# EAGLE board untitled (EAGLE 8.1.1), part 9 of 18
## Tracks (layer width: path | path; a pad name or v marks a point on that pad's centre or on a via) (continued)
S$8777 (continued)
  Bottom 0: 278.09,159.43 277.79,159.54
S$8778
  Bottom 0: 277.79,159.54 277.46,159.56
S$8779
  Bottom 0: 277.46,159.56 277.14,159.49
S$8780
  Bottom 0: 277.14,159.49 276.85,159.34
S$8781
  Bottom 0: 276.85,159.34 276.62,159.12
S$8782
  Bottom 0: 276.62,159.12 276.44,158.85
S$8783
  Bottom 0: 276.44,158.85 276.43,158.81
S$8784
  Bottom 0: 276.43,158.81 271.22,158.81
S$8785
  Bottom 0: 271.22,158.81 271.4,159.02
S$8786
  Bottom 0: 271.4,159.02 271.54,159.32
S$8787
  Bottom 0: 271.54,159.32 271.59,159.64
S$8788
  Bottom 0: 271.59,159.64 271.55,159.94
S$8789
  Bottom 0: 271.55,159.94 276.28,164.67
S$8790
  Bottom 0: 276.28,164.67 276.34,164.73
S$8791
  Bottom 0: 276.34,164.73 276.38,164.81
S$8792
  Bottom 0: 276.38,164.81 276.42,164.89
S$8793
  Bottom 0: 276.42,164.89 276.44,164.98
S$8794
  Bottom 0: 276.44,164.98 276.44,165.07
S$8795
  Bottom 0: 276.44,165.07 276.44,166.09
S$8796
  Bottom 0: 276.44,166.09 282.13,166.09
S$8797
  Bottom 0: 282.13,166.09 282.13,166.06
S$8798
  Bottom 0: 282.13,166.06 282.14,165.99
S$8799
  Bottom 0: 282.14,165.99 282.18,165.92
S$8800
  Bottom 0: 282.18,165.92 282.24,165.86
S$8801
  Bottom 0: 282.24,165.86 282.31,165.82
S$8802
  Bottom 0: 282.31,165.82 282.38,165.81
S$8803
  Bottom 0: 282.38,165.81 284.54,165.81
S$8804
  Bottom 0: 284.54,165.81 284.62,165.82
S$8805
  Bottom 0: 284.62,165.82 284.69,165.86
S$8806
  Bottom 0: 284.69,165.86 284.74,165.92
S$8807
  Bottom 0: 284.74,165.92 284.79,165.99
S$8808
  Bottom 0: 284.79,165.99 284.8,166.06
S$8809
  Bottom 0: 284.8,166.06 284.8,167.26
S$8810
  Bottom 0: 284.8,167.26 284.79,167.34
S$8811
  Bottom 0: 284.79,167.34 284.74,167.41
S$8812
  Bottom 0: 284.74,167.41 284.69,167.47
S$8813
  Bottom 0: 284.69,167.47 284.62,167.51
S$8814
  Bottom 0: 284.62,167.51 284.54,167.52
S$8815
  Bottom 0: 284.54,167.52 282.44,167.52
S$8816
  Bottom 0: 282.44,167.52 282.44,167.82
S$8817
  Bottom 0: 282.44,167.82 284.54,167.82
S$8818
  Bottom 0: 284.54,167.82 284.62,167.83
S$8819
  Bottom 0: 284.62,167.83 284.69,167.87
S$8820
  Bottom 0: 284.69,167.87 284.74,167.92
S$8821
  Bottom 0: 284.74,167.92 284.79,168
S$8822
  Bottom 0: 284.79,168 284.8,168.07
S$8823
  Bottom 0: 284.8,168.07 284.8,169.27
S$8824
  Bottom 0: 284.8,169.27 284.79,169.35
S$8825
  Bottom 0: 284.79,169.35 284.74,169.42
S$8826
  Bottom 0: 284.74,169.42 284.69,169.47
S$8827
  Bottom 0: 284.69,169.47 284.62,169.51
S$8828
  Bottom 0: 284.62,169.51 284.54,169.53
S$8829
  Bottom 0: 284.54,169.53 282.44,169.53
S$8830
  Bottom 0: 282.44,169.53 282.44,169.82
S$8831
  Bottom 0: 282.44,169.82 284.54,169.82
S$8832
  Bottom 0: 284.54,169.82 284.62,169.84
S$8833
  Bottom 0: 284.62,169.84 284.69,169.88
S$8834
  Bottom 0: 284.69,169.88 284.74,169.93
S$8835
  Bottom 0: 284.74,169.93 284.79,170
S$8836
  Bottom 0: 284.79,170 284.8,170.08
S$8837
  Bottom 0: 284.8,170.08 284.8,171.28
S$8838
  Bottom 0: 284.8,171.28 284.79,171.35
S$8839
  Bottom 0: 284.79,171.35 284.78,171.36
S$8840
  Bottom 0: 284.78,171.36 285.84,172.43
S$8841
  Bottom 0: 285.84,172.43 286.11,172.45
S$8842
  Bottom 0: 286.11,172.45 286.37,172.56
S$8843
  Bottom 0: 286.37,172.56 286.58,172.75
S$8844
  Bottom 0: 286.58,172.75 286.71,172.99
S$8845
  Bottom 0: 286.71,172.99 286.76,173.27
S$8846
  Bottom 0: 286.76,173.27 286.71,173.55
S$8847
  Bottom 0: 286.71,173.55 286.68,173.62
S$8848
  Bottom 0: 286.68,173.62 286.74,173.63
S$8849
  Bottom 0: 286.74,173.63 286.71,173.57
S$8850
  Bottom 0: 286.71,173.57 287.2,173.57
S$8851
  Bottom 0: 287.2,173.57 287.2,173.79
S$8852
  Bottom 0: 287.2,173.79 287.36,173.94
S$8853
  Bottom 0: 287.36,173.94 287.5,174.19
S$8854
  Bottom 0: 287.5,174.19 287.54,174.47
S$8855
  Bottom 0: 287.54,174.47 287.5,174.75
S$8856
  Bottom 0: 287.5,174.75 287.36,174.99
S$8857
  Bottom 0: 287.36,174.99 287.16,175.18
S$8858
  Bottom 0: 287.16,175.18 286.9,175.3
S$8859
  Bottom 0: 286.9,175.3 286.62,175.32
S$8860
  Bottom 0: 286.62,175.32 286.35,175.25
S$8861
  Bottom 0: 286.35,175.25 286.11,175.1
S$8862
  Bottom 0: 286.11,175.1 285.94,174.87
S$8863
  Bottom 0: 285.94,174.87 285.9,174.78
S$8864
  Bottom 0: 285.9,174.78 285.79,174.99
S$8865
  Bottom 0: 285.79,174.99 285.58,175.18
S$8866
  Bottom 0: 285.58,175.18 285.32,175.3
S$8867
  Bottom 0: 285.32,175.3 285.04,175.32
S$8868
  Bottom 0: 285.04,175.32 284.84,175.26
S$8869
  Bottom 0: 284.84,175.26 288.53,178.95
S$8870
  Bottom 0: 288.53,178.95 288.99,178.95
S$8871
  Bottom 0: 288.99,178.95 288.99,179.41
S$8872
  Bottom 0: 288.99,179.41 289.07,179.49
S$8873
  Bottom 0: 289.07,179.49 290.13,179.49
S$8874
  Bottom 0: 290.13,179.49 290.13,178.95
S$8875
  Bottom 0: 290.13,178.95 290.83,178.95
S$8876
  Bottom 0: 290.83,178.95 290.79,179.06
S$8877
  Bottom 0: 290.79,179.06 290.58,179.34
S$8878
  Bottom 0: 290.58,179.34 290.4,179.49
S$8879
  Bottom 0: 290.4,179.49 293.68,179.49
S$8880
  Bottom 0: 293.68,179.49 293.68,172.7
S$8881
  Bottom 0: 293.68,172.7 293.68,172.61
S$8882
  Bottom 0: 293.68,172.61 293.7,172.52
S$8883
  Bottom 0: 293.7,172.52 293.74,172.44
S$8884
  Bottom 0: 293.74,172.44 293.78,172.36
S$8885
  Bottom 0: 293.78,172.36 293.84,172.3
S$8886
  Bottom 0: 293.84,172.3 298.44,167.71
S$8887
  Bottom 0: 298.44,167.71 298.44,160.61
S$8888
  Bottom 0: 298.44,160.61 298.32,160.63
S$8889
  Bottom 0: 298.32,160.63 298.01,160.61
S$8890
  Bottom 0: 298.01,160.61 297.73,160.5
S$8891
  Bottom 0: 297.73,160.5 297.5,160.31
S$8892
  Bottom 0: 297.5,160.31 297.48,160.29
S$8893
  Bottom 0: 297.48,160.29 297.48,160.51
S$8894
  Bottom 0: 297.48,160.51 297.47,160.59
S$8895
  Bottom 0: 297.47,160.59 297.43,160.66
S$8896
  Bottom 0: 297.43,160.66 297.37,160.72
S$8897
  Bottom 0: 297.37,160.72 297.3,160.76
S$8898
  Bottom 0: 297.3,160.76 297.23,160.77
S$8899
  Bottom 0: 297.23,160.77 296.15,160.77
S$8900
  Bottom 0: 296.15,160.77 296.15,160.89
S$8901
  Bottom 0: 296.15,160.89 296.13,160.95
S$8902
  Bottom 0: 296.13,160.95 296.13,161.01
S$8903
  Bottom 0: 296.13,161.01 296.1,161.07
S$8904
  Bottom 0: 296.1,161.07 296.09,161.12
S$8905
  Bottom 0: 296.09,161.12 296.06,161.15
S$8906
  Bottom 0: 296.06,161.15 296.02,161.21
S$8907
  Bottom 0: 296.02,161.21 294.98,162.25
S$8908
  Bottom 0: 294.98,162.25 295,162.28
S$8909
  Bottom 0: 295,162.28 295.12,162.57
S$8910
  Bottom 0: 295.12,162.57 295.17,162.89
S$8911
  Bottom 0: 295.17,162.89 295.12,163.22
S$8912
  Bottom 0: 295.12,163.22 295,163.51
S$8913
  Bottom 0: 295,163.51 294.79,163.77
S$8914
  Bottom 0: 294.79,163.77 294.52,163.96
S$8915
  Bottom 0: 294.52,163.96 294.22,164.06
S$8916
  Bottom 0: 294.22,164.06 293.89,164.08
S$8917
  Bottom 0: 293.89,164.08 293.57,164.02
S$8918
  Bottom 0: 293.57,164.02 293.28,163.87
S$8919
  Bottom 0: 293.28,163.87 293.06,163.66
S$8920
  Bottom 0: 293.06,163.66 293.06,163.74
S$8921
  Bottom 0: 293.06,163.74 293.51,164.19
S$8922
  Bottom 0: 293.51,164.19 293.57,164.15
S$8923
  Bottom 0: 293.57,164.15 293.89,164.08
S$8924
  Bottom 0: 293.89,164.08 294.22,164.1
S$8925
  Bottom 0: 294.22,164.1 294.52,164.21
S$8926
  Bottom 0: 294.52,164.21 294.79,164.4
S$8927
  Bottom 0: 294.79,164.4 295,164.65
S$8928
  Bottom 0: 295,164.65 295.12,164.95
S$8929
  Bottom 0: 295.12,164.95 295.17,165.27
S$8930
  Bottom 0: 295.17,165.27 295.12,165.59
S$8931
  Bottom 0: 295.12,165.59 295,165.89
S$8932
  Bottom 0: 295,165.89 294.79,166.15
S$8933
  Bottom 0: 294.79,166.15 294.52,166.33
S$8934
  Bottom 0: 294.52,166.33 294.22,166.44
S$8935
  Bottom 0: 294.22,166.44 293.89,166.46
S$8936
  Bottom 0: 293.89,166.46 293.58,166.4
S$8937
  Bottom 0: 293.58,166.4 293.72,166.54
S$8938
  Bottom 0: 293.72,166.54 296.69,166.54
S$8939
  Bottom 0: 296.69,166.54 296.76,166.54
S$8940
  Bottom 0: 296.76,166.54 296.82,166.56
S$8941
  Bottom 0: 296.82,166.56 296.88,166.58
S$8942
  Bottom 0: 296.88,166.58 296.95,166.62
S$8943
  Bottom 0: 296.95,166.62 297,166.66
S$8944
  Bottom 0: 297,166.66 297.22,166.88
S$8945
  Bottom 0: 297.22,166.88 297.32,166.87
S$8946
  Bottom 0: 297.32,166.87 297.56,166.93
S$8947
  Bottom 0: 297.56,166.93 297.76,167.09
S$8948
  Bottom 0: 297.76,167.09 297.9,167.3
S$8949
  Bottom 0: 297.9,167.3 297.94,167.55
S$8950
  Bottom 0: 297.94,167.55 297.9,167.8
S$8951
  Bottom 0: 297.9,167.8 297.76,168.01
S$8952
  Bottom 0: 297.76,168.01 297.56,168.16
S$8953
  Bottom 0: 297.56,168.16 297.32,168.23
S$8954
  Bottom 0: 297.32,168.23 297.07,168.21
S$8955
  Bottom 0: 297.07,168.21 296.85,168.1
S$8956
  Bottom 0: 296.85,168.1 296.67,167.91
S$8957
  Bottom 0: 296.67,167.91 296.58,167.68
S$8958
  Bottom 0: 296.58,167.68 296.58,167.5
S$8959
  Bottom 0: 296.58,167.5 296.5,167.42
S$8960
  Bottom 0: 296.5,167.42 296.04,167.42
S$8961
  Bottom 0: 296.04,167.42 296.21,167.56
S$8962
  Bottom 0: 296.21,167.56 296.42,167.84
S$8963
  Bottom 0: 296.42,167.84 296.55,168.17
S$8964
  Bottom 0: 296.55,168.17 296.59,168.51
S$8965
  Bottom 0: 296.59,168.51 296.55,168.86
S$8966
  Bottom 0: 296.55,168.86 296.42,169.18
S$8967
  Bottom 0: 296.42,169.18 296.21,169.47
S$8968
  Bottom 0: 296.21,169.47 295.94,169.69
S$8969
  Bottom 0: 295.94,169.69 295.63,169.84
S$8970
  Bottom 0: 295.63,169.84 295.28,169.91
S$8971
  Bottom 0: 295.28,169.91 294.93,169.88
S$8972
  Bottom 0: 294.93,169.88 294.82,169.85
S$8973
  Bottom 0: 294.82,169.85 294.52,169.91
S$8974
  Bottom 0: 294.52,169.91 294.17,169.88
S$8975
  Bottom 0: 294.17,169.88 293.83,169.78
S$8976
  Bottom 0: 293.83,169.78 293.54,169.59
S$8977
  Bottom 0: 293.54,169.59 293.3,169.34
S$8978
  Bottom 0: 293.3,169.34 293.13,169.03
S$8979
  Bottom 0: 293.13,169.03 293.11,168.96
S$8980
  Bottom 0: 293.11,168.96 292.68,168.96
S$8981
  Bottom 0: 292.68,168.96 292.61,168.95
S$8982
  Bottom 0: 292.61,168.95 292.55,168.94
S$8983
  Bottom 0: 292.55,168.94 292.49,168.91
S$8984
  Bottom 0: 292.49,168.91 292.43,168.87
S$8985
  Bottom 0: 292.43,168.87 292.37,168.83
S$8986
  Bottom 0: 292.37,168.83 287.39,163.85
S$8987
  Bottom 0: 287.39,163.85 287.14,163.9
S$8988
  Bottom 0: 287.14,163.9 286.84,163.89
S$8989
  Bottom 0: 286.84,163.89 286.56,163.77
S$8990
  Bottom 0: 286.56,163.77 286.38,163.63
S$8991
  Bottom 0: 286.38,163.63 286.38,169.19
S$8992
  Bottom 0: 286.38,169.19 286.74,169.56
S$8993
  Bottom 0: 286.74,169.56 286.84,169.53
S$8994
  Bottom 0: 286.84,169.53 287.14,169.5
S$8995
  Bottom 0: 287.14,169.5 287.44,169.57
S$8996
  Bottom 0: 287.44,169.57 287.7,169.72
S$8997
  Bottom 0: 287.7,169.72 287.9,169.94
S$8998
  Bottom 0: 287.9,169.94 288.04,170.22
S$8999
  Bottom 0: 288.04,170.22 288.08,170.51
S$9000
  Bottom 0: 288.08,170.51 288.04,170.81
S$9001
  Bottom 0: 288.04,170.81 287.9,171.09
S$9002
  Bottom 0: 287.9,171.09 287.7,171.31
S$9003
  Bottom 0: 287.7,171.31 287.44,171.46
S$9004
  Bottom 0: 287.44,171.46 287.14,171.53
S$9005
  Bottom 0: 287.14,171.53 286.84,171.51
S$9006
  Bottom 0: 286.84,171.51 286.56,171.39
S$9007
  Bottom 0: 286.56,171.39 286.32,171.21
S$9008
  Bottom 0: 286.32,171.21 286.15,170.96
S$9009
  Bottom 0: 286.15,170.96 286.06,170.67
S$9010
  Bottom 0: 286.06,170.67 286.06,170.36
S$9011
  Bottom 0: 286.06,170.36 286.12,170.19
S$9012
  Bottom 0: 286.12,170.19 285.62,169.7
S$9013
  Bottom 0: 285.62,169.7 285.58,169.64
S$9014
  Bottom 0: 285.58,169.64 285.54,169.58
S$9015
  Bottom 0: 285.54,169.58 285.51,169.52
S$9016
  Bottom 0: 285.51,169.52 285.5,169.45
S$9017
  Bottom 0: 285.5,169.45 285.49,169.38
S$9018
  Bottom 0: 285.49,169.38 285.49,155.42
S$9019
  Bottom 0: 285.49,155.42 285,154.93
S$9020
  Bottom 0: 285,154.93 284.77,154.9
S$9021
  Bottom 0: 284.77,154.9 284.55,154.79
S$9022
  Bottom 0: 284.55,154.79 284.37,154.6
S$9023
  Bottom 0: 284.37,154.6 284.28,154.37
S$9024
  Bottom 0: 284.28,154.37 284.28,154.12
S$9025
  Bottom 0: 284.28,154.12 284.37,153.88
S$9026
  Bottom 0: 284.37,153.88 284.55,153.69
S$9027
  Bottom 0: 284.55,153.69 284.77,153.58
S$9028
  Bottom 0: 284.77,153.58 285.02,153.56
S$9029
  Bottom 0: 285.02,153.56 285.26,153.63
S$9030
  Bottom 0: 285.26,153.63 285.47,153.78
S$9031
  Bottom 0: 285.47,153.78 285.6,154
S$9032
  Bottom 0: 285.6,154 285.64,154.24
S$9033
  Bottom 0: 285.64,154.24 285.63,154.3
S$9034
  Bottom 0: 285.63,154.3 286.25,154.91
S$9035
  Bottom 0: 286.25,154.91 286.29,154.97
S$9036
  Bottom 0: 286.29,154.97 286.33,155.03
S$9037
  Bottom 0: 286.33,155.03 286.36,155.09
S$9038
  Bottom 0: 286.36,155.09 286.37,155.16
S$9039
  Bottom 0: 286.37,155.16 286.38,155.23
S$9040
  Bottom 0: 286.38,155.23 286.38,162.16
S$9041
  Bottom 0: 286.38,162.16 286.56,162.02
S$9042
  Bottom 0: 286.56,162.02 286.84,161.9
S$9043
  Bottom 0: 286.84,161.9 287.14,161.88
S$9044
  Bottom 0: 287.14,161.88 287.44,161.95
S$9045
  Bottom 0: 287.44,161.95 287.7,162.1
S$9046
  Bottom 0: 287.7,162.1 287.9,162.32
S$9047
  Bottom 0: 287.9,162.32 288.04,162.6
S$9048
  Bottom 0: 288.04,162.6 288.08,162.89
S$9049
  Bottom 0: 288.08,162.89 288.04,163.19
S$9050
  Bottom 0: 288.04,163.19 288.02,163.22
S$9051
  Bottom 0: 288.02,163.22 292.87,168.07
S$9052
  Bottom 0: 292.87,168.07 293.11,168.07
S$9053
  Bottom 0: 293.11,168.07 293.13,168
S$9054
  Bottom 0: 293.13,168 293.3,167.69
S$9055
  Bottom 0: 293.3,167.69 293.54,167.44
S$9056
  Bottom 0: 293.54,167.44 293.57,167.42
S$9057
  Bottom 0: 293.57,167.42 293.53,167.42
S$9058
  Bottom 0: 293.53,167.42 293.46,167.42
S$9059
  Bottom 0: 293.46,167.42 293.39,167.4
S$9060
  Bottom 0: 293.39,167.4 293.33,167.38
S$9061
  Bottom 0: 293.33,167.38 293.27,167.34
S$9062
  Bottom 0: 293.27,167.34 293.22,167.29
S$9063
  Bottom 0: 293.22,167.29 289.77,163.85
S$9064
  Bottom 0: 289.77,163.85 289.52,163.9
S$9065
  Bottom 0: 289.52,163.9 289.22,163.89
S$9066
  Bottom 0: 289.22,163.89 288.94,163.77
S$9067
  Bottom 0: 288.94,163.77 288.7,163.59
S$9068
  Bottom 0: 288.7,163.59 288.53,163.34
S$9069
  Bottom 0: 288.53,163.34 288.44,163.04
S$9070
  Bottom 0: 288.44,163.04 288.44,162.74
S$9071
  Bottom 0: 288.44,162.74 288.53,162.45
S$9072
  Bottom 0: 288.53,162.45 288.7,162.2
S$9073
  Bottom 0: 288.7,162.2 288.94,162.02
S$9074
  Bottom 0: 288.94,162.02 289.22,161.9
S$9075
  Bottom 0: 289.22,161.9 289.52,161.88
S$9076
  Bottom 0: 289.52,161.88 289.82,161.95
S$9077
  Bottom 0: 289.82,161.95 290.08,162.1
S$9078
  Bottom 0: 290.08,162.1 290.28,162.32
S$9079
  Bottom 0: 290.28,162.32 290.42,162.6
S$9080
  Bottom 0: 290.42,162.6 290.46,162.89
S$9081
  Bottom 0: 290.46,162.89 290.42,163.19
S$9082
  Bottom 0: 290.42,163.19 290.4,163.22
S$9083
  Bottom 0: 290.4,163.22 292.86,165.67
S$9084
  Bottom 0: 292.86,165.67 292.79,165.43
S$9085
  Bottom 0: 292.79,165.43 292.79,165.11
S$9086
  Bottom 0: 292.79,165.11 292.88,164.8
S$9087
  Bottom 0: 292.88,164.8 292.31,164.24
S$9088
  Bottom 0: 292.31,164.24 292.26,164.18
S$9089
  Bottom 0: 292.26,164.18 292.23,164.12
S$9090
  Bottom 0: 292.23,164.12 292.2,164.06
S$9091
  Bottom 0: 292.2,164.06 292.18,163.99
S$9092
  Bottom 0: 292.18,163.99 292.18,163.92
S$9093
  Bottom 0: 292.18,163.92 292.18,160.37
S$9094
  Bottom 0: 292.18,160.37 292.18,160.3
S$9095
  Bottom 0: 292.18,160.3 292.2,160.23
S$9096
  Bottom 0: 292.2,160.23 292.22,160.17
S$9097
  Bottom 0: 292.22,160.17 292.26,160.11
S$9098
  Bottom 0: 292.26,160.11 292.3,160.06
S$9099
  Bottom 0: 292.3,160.06 294.43,157.93
S$9100
  Bottom 0: 294.43,157.93 294.49,157.89
S$9101
  Bottom 0: 294.49,157.89 294.55,157.85
S$9102
  Bottom 0: 294.55,157.85 294.61,157.82
S$9103
  Bottom 0: 294.61,157.82 294.68,157.81
S$9104
  Bottom 0: 294.68,157.81 294.75,157.8
S$9105
  Bottom 0: 294.75,157.8 299.44,157.8
S$9106
  Bottom 0: 299.44,157.8 299.51,157.81
S$9107
  Bottom 0: 299.51,157.81 299.57,157.82
S$9108
  Bottom 0: 299.57,157.82 299.63,157.85
S$9109
  Bottom 0: 299.63,157.85 299.69,157.89
S$9110
  Bottom 0: 299.69,157.89 299.75,157.93
S$9111
  Bottom 0: 299.75,157.93 300.59,158.76
S$9112
  Bottom 0: 300.59,158.76 300.63,158.82
S$9113
  Bottom 0: 300.63,158.82 300.67,158.88
S$9114
  Bottom 0: 300.67,158.88 300.69,158.94
S$9115
  Bottom 0: 300.69,158.94 300.71,159.01
S$9116
  Bottom 0: 300.71,159.01 300.72,159.08
S$9117
  Bottom 0: 300.72,159.08 300.72,162.1
S$9118
  Bottom 0: 300.72,162.1 300.9,161.92
S$9119
  Bottom 0: 300.9,161.92 301.19,161.77
S$9120
  Bottom 0: 301.19,161.77 301.51,161.71
S$9121
  Bottom 0: 301.51,161.71 301.84,161.73
S$9122
  Bottom 0: 301.84,161.73 302.14,161.83
S$9123
  Bottom 0: 302.14,161.83 302.41,162.02
S$9124
  Bottom 0: 302.41,162.02 302.62,162.28
S$9125
  Bottom 0: 302.62,162.28 302.74,162.57
S$9126
  Bottom 0: 302.74,162.57 302.79,162.89
S$9127
  Bottom 0: 302.79,162.89 302.74,163.22
S$9128
  Bottom 0: 302.74,163.22 302.62,163.51
S$9129
  Bottom 0: 302.62,163.51 302.41,163.77
S$9130
  Bottom 0: 302.41,163.77 302.16,163.94
S$9131
  Bottom 0: 302.16,163.94 302.16,164.22
S$9132
  Bottom 0: 302.16,164.22 302.41,164.4
S$9133
  Bottom 0: 302.41,164.4 302.62,164.65
S$9134
  Bottom 0: 302.62,164.65 302.74,164.95
S$9135
  Bottom 0: 302.74,164.95 302.79,165.27
S$9136
  Bottom 0: 302.79,165.27 302.74,165.59
S$9137
  Bottom 0: 302.74,165.59 302.62,165.89
S$9138
  Bottom 0: 302.62,165.89 302.41,166.15
S$9139
  Bottom 0: 302.41,166.15 302.14,166.33
S$9140
  Bottom 0: 302.14,166.33 301.84,166.44
S$9141
  Bottom 0: 301.84,166.44 301.51,166.46
S$9142
  Bottom 0: 301.51,166.46 301.19,166.4
S$9143
  Bottom 0: 301.19,166.4 300.9,166.25
S$9144
  Bottom 0: 300.9,166.25 300.72,166.07
S$9145
  Bottom 0: 300.72,166.07 300.72,168.84
S$9146
  Bottom 0: 300.72,168.84 300.71,168.91
S$9147
  Bottom 0: 300.71,168.91 300.69,168.98
S$9148
  Bottom 0: 300.69,168.98 300.67,169.04
S$9149
  Bottom 0: 300.67,169.04 300.63,169.1
S$9150
  Bottom 0: 300.63,169.1 300.58,169.15
S$9151
  Bottom 0: 300.58,169.15 299.71,170.02
S$9152
  Bottom 0: 299.71,170.02 299.71,170.17
S$9153
  Bottom 0: 299.71,170.17 299.89,169.98
S$9154
  Bottom 0: 299.89,169.98 300.19,169.79
S$9155
  Bottom 0: 300.19,169.79 300.52,169.68
S$9156
  Bottom 0: 300.52,169.68 300.87,169.66
S$9157
  Bottom 0: 300.87,169.66 301.17,169.72
S$9158
  Bottom 0: 301.17,169.72 301.28,169.68
S$9159
  Bottom 0: 301.28,169.68 301.63,169.66
S$9160
  Bottom 0: 301.63,169.66 301.98,169.72
S$9161
  Bottom 0: 301.98,169.72 302.16,169.81
S$9162
  Bottom 0: 302.16,169.81 303.61,168.36
S$9163
  Bottom 0: 303.61,168.36 303.61,144.22
S$9164
  Bottom 0: 303.61,144.22 303.36,144.1
S$9165
  Bottom 0: 303.36,144.1 303.13,143.88
S$9166
  Bottom 0: 303.13,143.88 302.96,143.6
S$9167
  Bottom 0: 302.96,143.6 302.87,143.29
S$9168
  Bottom 0: 302.87,143.29 302.87,142.96
S$9169
  Bottom 0: 302.87,142.96 302.96,142.65
S$9170
  Bottom 0: 302.96,142.65 303.13,142.37
S$9171
  Bottom 0: 303.13,142.37 303.36,142.15
S$9172
  Bottom 0: 303.36,142.15 303.65,142
S$9173
  Bottom 0: 303.65,142 303.97,141.93
S$9174
  Bottom 0: 303.97,141.93 304.3,141.96
S$9175
  Bottom 0: 304.3,141.96 304.6,142.06
S$9176
  Bottom 0: 304.6,142.06 304.87,142.25
S$9177
  Bottom 0: 304.87,142.25 305.07,142.5
S$9178
  Bottom 0: 305.07,142.5 305.2,142.8
S$9179
  Bottom 0: 305.2,142.8 305.25,143.12
S$9180
  Bottom 0: 305.25,143.12 305.2,143.44
S$9181
  Bottom 0: 305.2,143.44 305.07,143.74
S$9182
  Bottom 0: 305.07,143.74 304.87,144
S$9183
  Bottom 0: 304.87,144 304.6,144.19
S$9184
  Bottom 0: 304.6,144.19 304.5,144.22
S$9185
  Bottom 0: 304.5,144.22 304.5,168.54
S$9186
  Bottom 0: 304.5,168.54 304.49,168.62
S$9187
  Bottom 0: 304.49,168.62 304.48,168.68
S$9188
  Bottom 0: 304.48,168.68 304.45,168.74
S$9189
  Bottom 0: 304.45,168.74 304.41,168.8
S$9190
  Bottom 0: 304.41,168.8 304.37,168.86
S$9191
  Bottom 0: 304.37,168.86 302.79,170.44
S$9192
  Bottom 0: 302.79,170.44 302.89,170.71
S$9193
  Bottom 0: 302.89,170.71 302.94,171.05
S$9194
  Bottom 0: 302.94,171.05 302.89,171.4
S$9195
  Bottom 0: 302.89,171.4 302.77,171.72
S$9196
  Bottom 0: 302.77,171.72 302.56,172.01
S$9197
  Bottom 0: 302.56,172.01 302.29,172.23
S$9198
  Bottom 0: 302.29,172.23 301.98,172.38
S$9199
  Bottom 0: 301.98,172.38 301.63,172.45
S$9200
  Bottom 0: 301.63,172.45 301.28,172.43
S$9201
  Bottom 0: 301.28,172.43 301.17,172.39
S$9202
  Bottom 0: 301.17,172.39 300.87,172.45
S$9203
  Bottom 0: 300.87,172.45 300.58,172.43
S$9204
  Bottom 0: 300.58,172.43 300.6,172.49
S$9205
  Bottom 0: 300.6,172.49 300.62,172.55
S$9206
  Bottom 0: 300.62,172.55 300.62,172.62
S$9207
  Bottom 0: 300.62,172.62 300.62,174.96
S$9208
  Bottom 0: 300.62,174.96 300.62,175.03
S$9209
  Bottom 0: 300.62,175.03 300.6,175.09
S$9210
  Bottom 0: 300.6,175.09 300.58,175.15
S$9211
  Bottom 0: 300.58,175.15 300.54,175.21
S$9212
  Bottom 0: 300.54,175.21 300.5,175.27
S$9213
  Bottom 0: 300.5,175.27 298.09,177.68
S$9214
  Bottom 0: 298.09,177.68 298.32,177.66
S$9215
  Bottom 0: 298.32,177.66 298.44,177.69
S$9216
  Bottom 0: 298.44,177.69 298.53,177.63
S$9217
  Bottom 0: 298.53,177.63 298.84,177.54
S$9218
  Bottom 0: 298.84,177.54 299.17,177.54
S$9219
  Bottom 0: 299.17,177.54 299.48,177.63
S$9220
  Bottom 0: 299.48,177.63 299.75,177.81
S$9221
  Bottom 0: 299.75,177.81 299.96,178.05
S$9222
  Bottom 0: 299.96,178.05 300.1,178.35
S$9223
  Bottom 0: 300.1,178.35 300.15,178.67
S$9224
  Bottom 0: 300.15,178.67 300.11,178.97
S$9225
  Bottom 0: 300.11,178.97 300.62,179.49
S$9226
  Bottom 0: 300.62,179.49 313.61,179.49
S$9227
  Bottom 0: 313.61,179.49 313.61,177.78
S$9228
  Bottom 0: 313.61,177.78 313.62,177.71
S$9229
  Bottom 0: 313.62,177.71 313.67,177.64
S$9230
  Bottom 0: 313.67,177.64 313.72,177.58
S$9231
  Bottom 0: 313.72,177.58 313.79,177.54
S$9232
  Bottom 0: 313.79,177.54 313.87,177.53
S$9233
  Bottom 0: 313.87,177.53 314.26,177.53
S$9234
  Bottom 0: 314.26,177.53 311.66,174.94
S$9235
  Bottom 0: 311.66,174.94 311.61,174.88
S$9236
  Bottom 0: 311.61,174.88 311.58,174.82
S$9237
  Bottom 0: 311.58,174.82 311.55,174.76
S$9238
  Bottom 0: 311.55,174.76 311.53,174.69
S$9239
  Bottom 0: 311.53,174.69 311.53,174.62
S$9240
  Bottom 0: 311.53,174.62 311.53,166.32
S$9241
  Bottom 0: 311.53,166.32 311.53,166.25
S$9242
  Bottom 0: 311.53,166.25 311.55,166.19
S$9243
  Bottom 0: 311.55,166.19 311.57,166.13
S$9244
  Bottom 0: 311.57,166.13 311.61,166.06
S$9245
  Bottom 0: 311.61,166.06 311.65,166.01
S$9246
  Bottom 0: 311.65,166.01 311.93,165.74
S$9247
  Bottom 0: 311.93,165.74 311.84,165.43
S$9248
  Bottom 0: 311.84,165.43 311.84,165.1
S$9249
  Bottom 0: 311.84,165.1 311.93,164.79
S$9250
  Bottom 0: 311.93,164.79 312.1,164.52
S$9251
  Bottom 0: 312.1,164.52 312.33,164.29
S$9252
  Bottom 0: 312.33,164.29 312.62,164.15
S$9253
  Bottom 0: 312.62,164.15 312.93,164.08
S$9254
  Bottom 0: 312.93,164.08 312.62,164.02
S$9255
  Bottom 0: 312.62,164.02 312.33,163.87
S$9256
  Bottom 0: 312.33,163.87 312.1,163.65
S$9257
  Bottom 0: 312.1,163.65 311.93,163.37
S$9258
  Bottom 0: 311.93,163.37 311.84,163.06
S$9259
  Bottom 0: 311.84,163.06 311.84,162.73
S$9260
  Bottom 0: 311.84,162.73 311.93,162.42
S$9261
  Bottom 0: 311.93,162.42 312.1,162.14
S$9262
  Bottom 0: 312.1,162.14 312.33,161.92
S$9263
  Bottom 0: 312.33,161.92 312.62,161.77
S$9264
  Bottom 0: 312.62,161.77 312.94,161.71
S$9265
  Bottom 0: 312.94,161.71 313.27,161.73
S$9266
  Bottom 0: 313.27,161.73 313.29,161.73
S$9267
  Bottom 0: 313.29,161.73 314.25,160.77
S$9268
  Bottom 0: 314.25,160.77 313.87,160.77
S$9269
  Bottom 0: 313.87,160.77 313.79,160.76
S$9270
  Bottom 0: 313.79,160.76 313.72,160.72
S$9271
  Bottom 0: 313.72,160.72 313.67,160.66
S$9272
  Bottom 0: 313.67,160.66 313.62,160.59
S$9273
  Bottom 0: 313.62,160.59 313.61,160.51
S$9274
  Bottom 0: 313.61,160.51 313.61,158.74
S$9275
  Bottom 0: 313.61,158.74 313.62,158.7
S$9276
  Bottom 0: 313.62,158.7 311.44,158.7
S$9277
  Bottom 0: 311.44,158.7 309.43,160.71
S$9278
  Bottom 0: 309.43,160.71 309.38,160.75
S$9279
  Bottom 0: 309.38,160.75 309.32,160.79
S$9280
  Bottom 0: 309.32,160.79 309.25,160.82
S$9281
  Bottom 0: 309.25,160.82 309.19,160.83
S$9282
  Bottom 0: 309.19,160.83 309.12,160.84
S$9283
  Bottom 0: 309.12,160.84 306.53,160.84
S$9284
  Bottom 0: 306.53,160.84 306.46,160.83
S$9285
  Bottom 0: 306.46,160.83 306.39,160.82
S$9286
  Bottom 0: 306.39,160.82 306.33,160.79
S$9287
  Bottom 0: 306.33,160.79 306.27,160.75
S$9288
  Bottom 0: 306.27,160.75 306.22,160.71
S$9289
  Bottom 0: 306.22,160.71 305.28,159.77
S$9290
  Bottom 0: 305.28,159.77 305.24,159.71
S$9291
  Bottom 0: 305.24,159.71 305.2,159.65
S$9292
  Bottom 0: 305.2,159.65 305.17,159.59
S$9293
  Bottom 0: 305.17,159.59 305.16,159.53
S$9294
  Bottom 0: 305.16,159.53 305.15,159.46
S$9295
  Bottom 0: 305.15,159.46 305.15,144.12
S$9296
  Bottom 0: 305.15,144.12 305.16,144.05
S$9297
  Bottom 0: 305.16,144.05 305.17,143.99
S$9298
  Bottom 0: 305.17,143.99 305.2,143.93
S$9299
  Bottom 0: 305.2,143.93 305.24,143.87
S$9300
  Bottom 0: 305.24,143.87 305.28,143.81
S$9301
  Bottom 0: 305.28,143.81 305.5,143.59
S$9302
  Bottom 0: 305.5,143.59 305.41,143.29
S$9303
  Bottom 0: 305.41,143.29 305.41,142.96
S$9304
  Bottom 0: 305.41,142.96 305.5,142.65
S$9305
  Bottom 0: 305.5,142.65 305.67,142.37
S$9306
  Bottom 0: 305.67,142.37 305.9,142.15
S$9307
  Bottom 0: 305.9,142.15 306.19,142
S$9308
  Bottom 0: 306.19,142 306.51,141.93
S$9309
  Bottom 0: 306.51,141.93 306.84,141.96
S$9310
  Bottom 0: 306.84,141.96 307.14,142.06
S$9311
  Bottom 0: 307.14,142.06 307.41,142.25
S$9312
  Bottom 0: 307.41,142.25 307.61,142.5
S$9313
  Bottom 0: 307.61,142.5 307.74,142.8
S$9314
  Bottom 0: 307.74,142.8 307.79,143.12
S$9315
  Bottom 0: 307.79,143.12 307.74,143.44
S$9316
  Bottom 0: 307.74,143.44 307.61,143.74
S$9317
  Bottom 0: 307.61,143.74 307.41,144
S$9318
  Bottom 0: 307.41,144 307.14,144.19
S$9319
  Bottom 0: 307.14,144.19 306.84,144.29
S$9320
  Bottom 0: 306.84,144.29 306.51,144.31
S$9321
  Bottom 0: 306.51,144.31 306.19,144.25
S$9322
  Bottom 0: 306.19,144.25 306.13,144.22
S$9323
  Bottom 0: 306.13,144.22 306.03,144.31
S$9324
  Bottom 0: 306.03,144.31 306.03,156.5
S$9325
  Bottom 0: 306.03,156.5 306.21,156.41
S$9326
  Bottom 0: 306.21,156.41 306.46,156.39
S$9327
  Bottom 0: 306.46,156.39 306.7,156.46
S$9328
  Bottom 0: 306.7,156.46 306.9,156.61
S$9329
  Bottom 0: 306.9,156.61 307.04,156.82
S$9330
  Bottom 0: 307.04,156.82 307.08,157.07
S$9331
  Bottom 0: 307.08,157.07 307.04,157.32
S$9332
  Bottom 0: 307.04,157.32 306.9,157.54
S$9333
  Bottom 0: 306.9,157.54 306.7,157.69
S$9334
  Bottom 0: 306.7,157.69 306.59,157.72
S$9335
  Bottom 0: 306.59,157.72 306.59,157.89
S$9336
  Bottom 0: 306.59,157.89 306.8,157.72
S$9337
  Bottom 0: 306.8,157.72 307.08,157.61
S$9338
  Bottom 0: 307.08,157.61 307.39,157.59
S$9339
  Bottom 0: 307.39,157.59 307.63,157.65
S$9340
  Bottom 0: 307.63,157.65 308.46,156.82
S$9341
  Bottom 0: 308.46,156.82 308.46,150.88
S$9342
  Bottom 0: 308.46,150.88 308.46,150.81
S$9343
  Bottom 0: 308.46,150.81 308.48,150.74
S$9344
  Bottom 0: 308.48,150.74 308.5,150.68
S$9345
  Bottom 0: 308.5,150.68 308.54,150.62
S$9346
  Bottom 0: 308.54,150.62 308.58,150.57
S$9347
  Bottom 0: 308.58,150.57 309.01,150.14
S$9348
  Bottom 0: 309.01,150.14 308.85,150.12
S$9349
  Bottom 0: 308.85,150.12 308.81,150.11
S$9350
  Bottom 0: 308.81,150.11 308.26,150.66
S$9351
  Bottom 0: 308.26,150.66 308.28,150.68
S$9352
  Bottom 0: 308.28,150.68 308.33,150.98
S$9353
  Bottom 0: 308.33,150.98 308.28,151.28
S$9354
  Bottom 0: 308.28,151.28 308.15,151.56
S$9355
  Bottom 0: 308.15,151.56 307.94,151.78
S$9356
  Bottom 0: 307.94,151.78 307.68,151.93
S$9357
  Bottom 0: 307.68,151.93 307.39,151.99
S$9358
  Bottom 0: 307.39,151.99 307.08,151.97
S$9359
  Bottom 0: 307.08,151.97 306.8,151.86
S$9360
  Bottom 0: 306.8,151.86 306.56,151.67
S$9361
  Bottom 0: 306.56,151.67 306.39,151.43
S$9362
  Bottom 0: 306.39,151.43 306.3,151.13
S$9363
  Bottom 0: 306.3,151.13 306.3,150.83
S$9364
  Bottom 0: 306.3,150.83 306.39,150.54
S$9365
  Bottom 0: 306.39,150.54 306.56,150.29
S$9366
  Bottom 0: 306.56,150.29 306.8,150.1
S$9367
  Bottom 0: 306.8,150.1 307.08,149.99
S$9368
  Bottom 0: 307.08,149.99 307.39,149.97
S$9369
  Bottom 0: 307.39,149.97 307.63,150.03
S$9370
  Bottom 0: 307.63,150.03 308.38,149.28
S$9371
  Bottom 0: 308.38,149.28 308.45,149.1
S$9372
  Bottom 0: 308.45,149.1 308.62,148.91
S$9373
  Bottom 0: 308.62,148.91 308.85,148.8
S$9374
  Bottom 0: 308.85,148.8 309.1,148.78
S$9375
  Bottom 0: 309.1,148.78 309.34,148.85
S$9376
  Bottom 0: 309.34,148.85 309.55,149
S$9377
  Bottom 0: 309.55,149 309.68,149.22
S$9378
  Bottom 0: 309.68,149.22 309.71,149.43
S$9379
  Bottom 0: 309.71,149.43 315.14,144
S$9380
  Bottom 0: 315.14,144 315.14,143.85
S$9381
  Bottom 0: 315.14,143.85 315.03,144
S$9382
  Bottom 0: 315.03,144 314.76,144.19
S$9383
  Bottom 0: 314.76,144.19 314.46,144.29
S$9384
  Bottom 0: 314.46,144.29 314.13,144.31
S$9385
  Bottom 0: 314.13,144.31 313.81,144.25
S$9386
  Bottom 0: 313.81,144.25 313.52,144.1
S$9387
  Bottom 0: 313.52,144.1 313.29,143.88
S$9388
  Bottom 0: 313.29,143.88 313.12,143.6
S$9389
  Bottom 0: 313.12,143.6 313.03,143.29
S$9390
  Bottom 0: 313.03,143.29 313.03,142.96
S$9391
  Bottom 0: 313.03,142.96 313.12,142.65
S$9392
  Bottom 0: 313.12,142.65 313.29,142.37
S$9393
  Bottom 0: 313.29,142.37 313.52,142.15
S$9394
  Bottom 0: 313.52,142.15 313.81,142
S$9395
  Bottom 0: 313.81,142 314.13,141.93
S$9396
  Bottom 0: 314.13,141.93 314.46,141.96
S$9397
  Bottom 0: 314.46,141.96 314.76,142.06
S$9398
  Bottom 0: 314.76,142.06 315.03,142.25
S$9399
  Bottom 0: 315.03,142.25 315.14,142.39
S$9400
  Bottom 0: 315.14,142.39 315.14,137.07
S$9401
  Bottom 0: 315.14,137.07 307.06,128.98
S$9402
  Bottom 0: 307.06,128.98 306.84,129.05
S$9403
  Bottom 0: 306.84,129.05 306.51,129.07
S$9404
  Bottom 0: 306.51,129.07 306.19,129.01
S$9405
  Bottom 0: 306.19,129.01 305.9,128.86
S$9406
  Bottom 0: 305.9,128.86 305.67,128.64
S$9407
  Bottom 0: 305.67,128.64 305.5,128.36
S$9408
  Bottom 0: 305.5,128.36 305.41,128.05
S$9409
  Bottom 0: 305.41,128.05 305.41,127.72
S$9410
  Bottom 0: 305.41,127.72 305.5,127.41
S$9411
  Bottom 0: 305.5,127.41 305.67,127.13
S$9412
  Bottom 0: 305.67,127.13 305.9,126.91
S$9413
  Bottom 0: 305.9,126.91 306.19,126.76
S$9414
  Bottom 0: 306.19,126.76 306.51,126.69
S$9415
  Bottom 0: 306.51,126.69 306.84,126.72
S$9416
  Bottom 0: 306.84,126.72 307.14,126.82
S$9417
  Bottom 0: 307.14,126.82 307.41,127.01
S$9418
  Bottom 0: 307.41,127.01 307.61,127.26
S$9419
  Bottom 0: 307.61,127.26 307.74,127.56
S$9420
  Bottom 0: 307.74,127.56 307.79,127.88
S$9421
  Bottom 0: 307.79,127.88 307.74,128.2
S$9422
  Bottom 0: 307.74,128.2 307.68,128.34
S$9423
  Bottom 0: 307.68,128.34 315.71,136.37
S$9424
  Bottom 0: 315.71,136.37 315.71,132.54
S$9425
  Bottom 0: 315.71,132.54 312.14,128.98
S$9426
  Bottom 0: 312.14,128.98 311.92,129.05
S$9427
  Bottom 0: 311.92,129.05 311.59,129.07
S$9428
  Bottom 0: 311.59,129.07 311.27,129.01
S$9429
  Bottom 0: 311.27,129.01 310.98,128.86
S$9430
  Bottom 0: 310.98,128.86 310.75,128.64
S$9431
  Bottom 0: 310.75,128.64 310.58,128.36
S$9432
  Bottom 0: 310.58,128.36 310.49,128.05
S$9433
  Bottom 0: 310.49,128.05 310.49,127.72
S$9434
  Bottom 0: 310.49,127.72 310.58,127.41
S$9435
  Bottom 0: 310.58,127.41 310.75,127.13
S$9436
  Bottom 0: 310.75,127.13 310.98,126.91
S$9437
  Bottom 0: 310.98,126.91 311.27,126.76
S$9438
  Bottom 0: 311.27,126.76 311.59,126.69
S$9439
  Bottom 0: 311.59,126.69 311.92,126.72
S$9440
  Bottom 0: 311.92,126.72 312.22,126.82
S$9441
  Bottom 0: 312.22,126.82 312.49,127.01
S$9442
  Bottom 0: 312.49,127.01 312.69,127.26
S$9443
  Bottom 0: 312.69,127.26 312.82,127.56
S$9444
  Bottom 0: 312.82,127.56 312.87,127.88
S$9445
  Bottom 0: 312.87,127.88 312.82,128.2
S$9446
  Bottom 0: 312.82,128.2 312.76,128.35
S$9447
  Bottom 0: 312.76,128.35 316.4,131.99
S$9448
  Bottom 0: 316.4,131.99 316.4,130.7
S$9449
  Bottom 0: 316.4,130.7 314.68,128.98
S$9450
  Bottom 0: 314.68,128.98 314.46,129.05
S$9451
  Bottom 0: 314.46,129.05 314.13,129.07
S$9452
  Bottom 0: 314.13,129.07 313.81,129.01
S$9453
  Bottom 0: 313.81,129.01 313.52,128.86
S$9454
  Bottom 0: 313.52,128.86 313.29,128.64
S$9455
  Bottom 0: 313.29,128.64 313.12,128.36
S$9456
  Bottom 0: 313.12,128.36 313.03,128.05
S$9457
  Bottom 0: 313.03,128.05 313.03,127.72
S$9458
  Bottom 0: 313.03,127.72 313.12,127.41
S$9459
  Bottom 0: 313.12,127.41 313.29,127.13
S$9460
  Bottom 0: 313.29,127.13 313.52,126.91
S$9461
  Bottom 0: 313.52,126.91 313.81,126.76
S$9462
  Bottom 0: 313.81,126.76 314.13,126.69
S$9463
  Bottom 0: 314.13,126.69 314.46,126.72
S$9464
  Bottom 0: 314.46,126.72 314.76,126.82
S$9465
  Bottom 0: 314.76,126.82 315.03,127.01
S$9466
  Bottom 0: 315.03,127.01 315.23,127.26
S$9467
  Bottom 0: 315.23,127.26 315.36,127.56
S$9468
  Bottom 0: 315.36,127.56 315.41,127.88
S$9469
  Bottom 0: 315.41,127.88 315.36,128.2
S$9470
  Bottom 0: 315.36,128.2 315.3,128.35
S$9471
  Bottom 0: 315.3,128.35 317.16,130.21
S$9472
  Bottom 0: 317.16,130.21 317.2,130.26
S$9473
  Bottom 0: 317.2,130.26 317.24,130.32
S$9474
  Bottom 0: 317.24,130.32 317.27,130.38
S$9475
  Bottom 0: 317.27,130.38 317.28,130.45
S$9476
  Bottom 0: 317.28,130.45 317.29,130.52
S$9477
  Bottom 0: 317.29,130.52 317.29,150.99
S$9478
  Bottom 0: 317.29,150.99 318.45,152.15
S$9479
  Bottom 0: 318.45,152.15 318.45,151.83
S$9480
  Bottom 0: 318.45,151.83 318.54,151.49
S$9481
  Bottom 0: 318.54,151.49 318.71,151.18
S$9482
  Bottom 0: 318.71,151.18 318.95,150.93
S$9483
  Bottom 0: 318.95,150.93 319.24,150.74
S$9484
  Bottom 0: 319.24,150.74 319.57,150.63
S$9485
  Bottom 0: 319.57,150.63 319.92,150.61
S$9486
  Bottom 0: 319.92,150.61 320.23,150.67
S$9487
  Bottom 0: 320.23,150.67 320.33,150.63
S$9488
  Bottom 0: 320.33,150.63 320.69,150.61
S$9489
  Bottom 0: 320.69,150.61 321.03,150.67
S$9490
  Bottom 0: 321.03,150.67 321.21,150.76
S$9491
  Bottom 0: 321.21,150.76 321.52,150.45
S$9492
  Bottom 0: 321.52,150.45 321.52,144.4
S$9493
  Bottom 0: 321.52,144.4 320.62,144.4
S$9494
  Bottom 0: 320.62,144.4 320.54,144.39
S$9495
  Bottom 0: 320.54,144.39 320.47,144.35
S$9496
  Bottom 0: 320.47,144.35 320.42,144.3
S$9497
  Bottom 0: 320.42,144.3 320.38,144.22
S$9498
  Bottom 0: 320.38,144.22 320.37,144.15
S$9499
  Bottom 0: 320.37,144.15 320.37,116.33
S$9500
  Bottom 0: 320.37,116.33 320.38,116.25
S$9501
  Bottom 0: 320.38,116.25 320.42,116.18
S$9502
  Bottom 0: 320.42,116.18 320.47,116.12
S$9503
  Bottom 0: 320.47,116.12 320.54,116.08
S$9504
  Bottom 0: 320.54,116.08 320.62,116.07
S$9505
  Bottom 0: 320.62,116.07 321.52,116.07
S$9506
  Bottom 0: 321.52,116.07 321.52,106.54
S$9507
  Bottom 0: 321.52,106.54 321.46,106.62
S$9508
  Bottom 0: 321.46,106.62 321.19,106.81
S$9509
  Bottom 0: 321.19,106.81 320.89,106.91
S$9510
  Bottom 0: 320.89,106.91 320.56,106.93
S$9511
  Bottom 0: 320.56,106.93 320.31,106.88
S$9512
  Bottom 0: 320.31,106.88 319.44,107.75
S$9513
  Bottom 0: 319.44,107.75 319.38,107.81
S$9514
  Bottom 0: 319.38,107.81 319.3,107.86
S$9515
  Bottom 0: 319.3,107.86 319.22,107.89
S$9516
  Bottom 0: 319.22,107.89 319.13,107.91
S$9517
  Bottom 0: 319.13,107.91 319.04,107.92
S$9518
  Bottom 0: 319.04,107.92 303.77,107.92
S$9519
  Bottom 0: 303.77,107.92 303.77,119.86
S$9520
  Bottom 0: 303.77,119.86 303.89,119.8
S$9521
  Bottom 0: 303.89,119.8 304.14,119.78
S$9522
  Bottom 0: 304.14,119.78 304.38,119.84
S$9523
  Bottom 0: 304.38,119.84 304.59,120
S$9524
  Bottom 0: 304.59,120 304.72,120.21
S$9525
  Bottom 0: 304.72,120.21 304.76,120.46
S$9526
  Bottom 0: 304.76,120.46 304.72,120.71
S$9527
  Bottom 0: 304.72,120.71 304.59,120.92
S$9528
  Bottom 0: 304.59,120.92 304.52,120.97
S$9529
  Bottom 0: 304.52,120.97 304.52,124.16
S$9530
  Bottom 0: 304.52,124.16 304.52,124.23
S$9531
  Bottom 0: 304.52,124.23 304.5,124.29
S$9532
  Bottom 0: 304.5,124.29 304.48,124.35
S$9533
  Bottom 0: 304.48,124.35 304.43,124.41
S$9534
  Bottom 0: 304.43,124.41 304.39,124.47
S$9535
  Bottom 0: 304.39,124.47 302.45,126.42
S$9536
  Bottom 0: 302.45,126.42 302.39,126.46
S$9537
  Bottom 0: 302.39,126.46 302.33,126.5
S$9538
  Bottom 0: 302.33,126.5 302.27,126.52
S$9539
  Bottom 0: 302.27,126.52 302.2,126.54
S$9540
  Bottom 0: 302.2,126.54 302.13,126.54
S$9541
  Bottom 0: 302.13,126.54 300.94,126.54
S$9542
  Bottom 0: 300.94,126.54 300.06,127.43
S$9543
  Bottom 0: 300.06,127.43 300.12,127.56
S$9544
  Bottom 0: 300.12,127.56 300.17,127.88
S$9545
  Bottom 0: 300.17,127.88 300.12,128.2
S$9546
  Bottom 0: 300.12,128.2 299.99,128.5
S$9547
  Bottom 0: 299.99,128.5 299.79,128.76
S$9548
  Bottom 0: 299.79,128.76 299.52,128.95
S$9549
  Bottom 0: 299.52,128.95 299.22,129.05
S$9550
  Bottom 0: 299.22,129.05 298.89,129.07
S$9551
  Bottom 0: 298.89,129.07 298.57,129.01
S$9552
  Bottom 0: 298.57,129.01 298.28,128.86
S$9553
  Bottom 0: 298.28,128.86 298.05,128.64
S$9554
  Bottom 0: 298.05,128.64 297.88,128.36
S$9555
  Bottom 0: 297.88,128.36 297.79,128.05
S$9556
  Bottom 0: 297.79,128.05 297.79,127.72
S$9557
  Bottom 0: 297.79,127.72 297.88,127.41
S$9558
  Bottom 0: 297.88,127.41 298.05,127.13
S$9559
  Bottom 0: 298.05,127.13 298.28,126.91
S$9560
  Bottom 0: 298.28,126.91 298.57,126.76
S$9561
  Bottom 0: 298.57,126.76 298.89,126.69
S$9562
  Bottom 0: 298.89,126.69 299.22,126.72
S$9563
  Bottom 0: 299.22,126.72 299.44,126.79
S$9564
  Bottom 0: 299.44,126.79 300.44,125.79
S$9565
  Bottom 0: 300.44,125.79 300.5,125.75
S$9566
  Bottom 0: 300.5,125.75 300.56,125.7
S$9567
  Bottom 0: 300.56,125.7 300.62,125.68
S$9568
  Bottom 0: 300.62,125.68 300.69,125.66
S$9569
  Bottom 0: 300.69,125.66 300.76,125.66
S$9570
  Bottom 0: 300.76,125.66 300.79,125.66
S$9571
  Bottom 0: 300.79,125.66 300.67,125.54
S$9572
  Bottom 0: 300.67,125.54 300.5,125.27
S$9573
  Bottom 0: 300.5,125.27 300.41,124.95
S$9574
  Bottom 0: 300.41,124.95 300.41,124.63
S$9575
  Bottom 0: 300.41,124.63 300.44,124.5
S$9576
  Bottom 0: 300.44,124.5 297.52,127.43
S$9577
  Bottom 0: 297.52,127.43 297.58,127.56
S$9578
  Bottom 0: 297.58,127.56 297.63,127.88
S$9579
  Bottom 0: 297.63,127.88 297.58,128.2
S$9580
  Bottom 0: 297.58,128.2 297.45,128.5
S$9581
  Bottom 0: 297.45,128.5 297.25,128.76
S$9582
  Bottom 0: 297.25,128.76 296.98,128.95
S$9583
  Bottom 0: 296.98,128.95 296.68,129.05
S$9584
  Bottom 0: 296.68,129.05 296.35,129.07
S$9585
  Bottom 0: 296.35,129.07 296.03,129.01
S$9586
  Bottom 0: 296.03,129.01 295.74,128.86
S$9587
  Bottom 0: 295.74,128.86 295.51,128.64
S$9588
  Bottom 0: 295.51,128.64 295.34,128.36
S$9589
  Bottom 0: 295.34,128.36 295.25,128.05
S$9590
  Bottom 0: 295.25,128.05 295.25,127.72
S$9591
  Bottom 0: 295.25,127.72 295.34,127.41
S$9592
  Bottom 0: 295.34,127.41 295.51,127.13
S$9593
  Bottom 0: 295.51,127.13 295.74,126.91
S$9594
  Bottom 0: 295.74,126.91 296.03,126.76
S$9595
  Bottom 0: 296.03,126.76 296.15,126.74
S$9596
  Bottom 0: 296.15,126.74 296.09,126.74
S$9597
  Bottom 0: 296.09,126.74 294.21,126.74
S$9598
  Bottom 0: 294.21,126.74 294.44,126.82
S$9599
  Bottom 0: 294.44,126.82 294.71,127.01
S$9600
  Bottom 0: 294.71,127.01 294.91,127.26
S$9601
  Bottom 0: 294.91,127.26 295.04,127.56
S$9602
  Bottom 0: 295.04,127.56 295.09,127.88
S$9603
  Bottom 0: 295.09,127.88 295.04,128.2
S$9604
  Bottom 0: 295.04,128.2 294.91,128.5
S$9605
  Bottom 0: 294.91,128.5 294.71,128.76
S$9606
  Bottom 0: 294.71,128.76 294.44,128.95
S$9607
  Bottom 0: 294.44,128.95 294.14,129.05
S$9608
  Bottom 0: 294.14,129.05 293.81,129.07
S$9609
  Bottom 0: 293.81,129.07 293.49,129.01
S$9610
  Bottom 0: 293.49,129.01 293.2,128.86
S$9611
  Bottom 0: 293.2,128.86 292.97,128.64
S$9612
  Bottom 0: 292.97,128.64 292.8,128.36
S$9613
  Bottom 0: 292.8,128.36 292.71,128.05
S$9614
  Bottom 0: 292.71,128.05 292.71,127.72
S$9615
  Bottom 0: 292.71,127.72 292.8,127.41
S$9616
  Bottom 0: 292.8,127.41 292.97,127.13
S$9617
  Bottom 0: 292.97,127.13 293.2,126.91
S$9618
  Bottom 0: 293.2,126.91 293.49,126.76
S$9619
  Bottom 0: 293.49,126.76 293.59,126.74
S$9620
  Bottom 0: 293.59,126.74 293.13,126.74
S$9621
  Bottom 0: 293.13,126.74 292.44,127.43
S$9622
  Bottom 0: 292.44,127.43 292.5,127.56
S$9623
  Bottom 0: 292.5,127.56 292.55,127.88
S$9624
  Bottom 0: 292.55,127.88 292.5,128.2
S$9625
  Bottom 0: 292.5,128.2 292.37,128.5
S$9626
  Bottom 0: 292.37,128.5 292.17,128.76
S$9627
  Bottom 0: 292.17,128.76 291.9,128.95
S$9628
  Bottom 0: 291.9,128.95 291.6,129.05
S$9629
  Bottom 0: 291.6,129.05 291.27,129.07
S$9630
  Bottom 0: 291.27,129.07 290.95,129.01
S$9631
  Bottom 0: 290.95,129.01 290.66,128.86
S$9632
  Bottom 0: 290.66,128.86 290.43,128.64
S$9633
  Bottom 0: 290.43,128.64 290.26,128.36
S$9634
  Bottom 0: 290.26,128.36 290.17,128.05
S$9635
  Bottom 0: 290.17,128.05 290.17,127.72
S$9636
  Bottom 0: 290.17,127.72 290.26,127.41
S$9637
  Bottom 0: 290.26,127.41 290.43,127.13
S$9638
  Bottom 0: 290.43,127.13 290.66,126.91
S$9639
  Bottom 0: 290.66,126.91 290.95,126.76
S$9640
  Bottom 0: 290.95,126.76 291.27,126.69
S$9641
  Bottom 0: 291.27,126.69 291.6,126.72
S$9642
  Bottom 0: 291.6,126.72 291.82,126.79
S$9643
  Bottom 0: 291.82,126.79 292.62,125.98
S$9644
  Bottom 0: 292.62,125.98 292.68,125.94
S$9645
  Bottom 0: 292.68,125.94 292.74,125.9
S$9646
  Bottom 0: 292.74,125.9 292.8,125.88
S$9647
  Bottom 0: 292.8,125.88 292.87,125.86
S$9648
  Bottom 0: 292.87,125.86 292.94,125.86
S$9649
  Bottom 0: 292.94,125.86 293.46,125.86
S$9650
  Bottom 0: 293.46,125.86 293.28,125.77
S$9651
  Bottom 0: 293.28,125.77 293.05,125.54
S$9652
  Bottom 0: 293.05,125.54 292.88,125.27
S$9653
  Bottom 0: 292.88,125.27 292.79,124.95
S$9654
  Bottom 0: 292.79,124.95 292.79,124.63
S$9655
  Bottom 0: 292.79,124.63 292.88,124.31
S$9656
  Bottom 0: 292.88,124.31 293.05,124.04
S$9657
  Bottom 0: 293.05,124.04 293.28,123.81
S$9658
  Bottom 0: 293.28,123.81 293.57,123.67
S$9659
  Bottom 0: 293.57,123.67 293.89,123.6
S$9660
  Bottom 0: 293.89,123.6 294.22,123.62
S$9661
  Bottom 0: 294.22,123.62 294.52,123.73
S$9662
  Bottom 0: 294.52,123.73 294.79,123.92
S$9663
  Bottom 0: 294.79,123.92 295,124.17
S$9664
  Bottom 0: 295,124.17 295.12,124.47
S$9665
  Bottom 0: 295.12,124.47 295.17,124.79
S$9666
  Bottom 0: 295.17,124.79 295.12,125.11
S$9667
  Bottom 0: 295.12,125.11 295,125.41
S$9668
  Bottom 0: 295,125.41 294.79,125.66
S$9669
  Bottom 0: 294.79,125.66 294.52,125.85
S$9670
  Bottom 0: 294.52,125.85 294.51,125.86
S$9671
  Bottom 0: 294.51,125.86 295.9,125.86
S$9672
  Bottom 0: 295.9,125.86 298.69,123.07
S$9673
  Bottom 0: 298.69,123.07 298.69,122.89
S$9674
  Bottom 0: 298.69,122.89 298.79,122.66
S$9675
  Bottom 0: 298.79,122.66 298.8,122.64
S$9676
  Bottom 0: 298.8,122.64 298.64,122.59
S$9677
  Bottom 0: 298.64,122.59 297.83,123.39
S$9678
  Bottom 0: 297.83,123.39 297.77,123.45
S$9679
  Bottom 0: 297.77,123.45 297.69,123.5
S$9680
  Bottom 0: 297.69,123.5 297.61,123.53
S$9681
  Bottom 0: 297.61,123.53 297.52,123.56
S$9682
  Bottom 0: 297.52,123.56 297.43,123.56
S$9683
  Bottom 0: 297.43,123.56 287.54,123.56
S$9684
  Bottom 0: 287.54,123.56 287.54,127.19
S$9685
  Bottom 0: 287.54,127.19 287.53,127.28
S$9686
  Bottom 0: 287.53,127.28 287.51,127.37
S$9687
  Bottom 0: 287.51,127.37 287.48,127.45
S$9688
  Bottom 0: 287.48,127.45 287.43,127.52
S$9689
  Bottom 0: 287.43,127.52 287.41,127.54
S$9690
  Bottom 0: 287.41,127.54 287.42,127.56
S$9691
  Bottom 0: 287.42,127.56 287.47,127.88
S$9692
  Bottom 0: 287.47,127.88 287.42,128.2
S$9693
  Bottom 0: 287.42,128.2 287.29,128.5
S$9694
  Bottom 0: 287.29,128.5 287.09,128.76
S$9695
  Bottom 0: 287.09,128.76 286.82,128.95
S$9696
  Bottom 0: 286.82,128.95 286.52,129.05
S$9697
  Bottom 0: 286.52,129.05 286.19,129.07
S$9698
  Bottom 0: 286.19,129.07 285.87,129.01
S$9699
  Bottom 0: 285.87,129.01 285.58,128.86
S$9700
  Bottom 0: 285.58,128.86 285.35,128.64
S$9701
  Bottom 0: 285.35,128.64 285.18,128.36
S$9702
  Bottom 0: 285.18,128.36 285.09,128.05
S$9703
  Bottom 0: 285.09,128.05 285.09,127.72
S$9704
  Bottom 0: 285.09,127.72 285.18,127.41
S$9705
  Bottom 0: 285.18,127.41 285.35,127.13
S$9706
  Bottom 0: 285.35,127.13 285.58,126.91
S$9707
  Bottom 0: 285.58,126.91 285.87,126.76
S$9708
  Bottom 0: 285.87,126.76 286.19,126.69
S$9709
  Bottom 0: 286.19,126.69 286.4,126.71
S$9710
  Bottom 0: 286.4,126.71 286.4,103.71
S$9711
  Bottom 0: 286.4,103.71 285.55,102.86
S$9712
  Bottom 0: 285.55,102.86 281.03,102.86
S$9713
  Bottom 0: 281.03,102.86 280.92,103.09
S$9714
  Bottom 0: 280.92,103.09 280.71,103.34
S$9715
  Bottom 0: 280.71,103.34 280.44,103.52
S$9716
  Bottom 0: 280.44,103.52 280.12,103.61
S$9717
  Bottom 0: 280.12,103.61 279.8,103.61
S$9718
  Bottom 0: 279.8,103.61 279.49,103.52
S$9719
  Bottom 0: 279.49,103.52 279.4,103.46
S$9720
  Bottom 0: 279.4,103.46 279.28,103.48
S$9721
  Bottom 0: 279.28,103.48 278.97,103.46
S$9722
  Bottom 0: 278.97,103.46 278.69,103.35
S$9723
  Bottom 0: 278.69,103.35 278.45,103.17
S$9724
  Bottom 0: 278.45,103.17 278.43,103.13
S$9725
  Bottom 0: 278.43,103.13 278.43,103.37
S$9726
  Bottom 0: 278.43,103.37 278.42,103.44
S$9727
  Bottom 0: 278.42,103.44 278.38,103.52
S$9728
  Bottom 0: 278.38,103.52 278.32,103.57
S$9729
  Bottom 0: 278.32,103.57 278.25,103.61
S$9730
  Bottom 0: 278.25,103.61 278.18,103.62
S$9731
  Bottom 0: 278.18,103.62 277.1,103.62
S$9732
  Bottom 0: 277.1,103.62 277.1,103.74
S$9733
  Bottom 0: 277.1,103.74 277.08,103.8
S$9734
  Bottom 0: 277.08,103.8 277.08,103.86
S$9735
  Bottom 0: 277.08,103.86 277.05,103.93
S$9736
  Bottom 0: 277.05,103.93 277.04,103.97
S$9737
  Bottom 0: 277.04,103.97 277.01,104
S$9738
  Bottom 0: 277.01,104 276.97,104.06
S$9739
  Bottom 0: 276.97,104.06 275.93,105.1
S$9740
  Bottom 0: 275.93,105.1 275.94,105.11
S$9741
  Bottom 0: 275.94,105.11 276.07,105.42
S$9742
  Bottom 0: 276.07,105.42 276.11,105.73
S$9743
  Bottom 0: 276.11,105.73 276.07,106.06
S$9744
  Bottom 0: 276.07,106.06 275.94,106.36
S$9745
  Bottom 0: 275.94,106.36 275.73,106.61
S$9746
  Bottom 0: 275.73,106.61 275.47,106.8
S$9747
  Bottom 0: 275.47,106.8 275.16,106.9
S$9748
  Bottom 0: 275.16,106.9 274.84,106.92
S$9749
  Bottom 0: 274.84,106.92 274.52,106.86
S$9750
  Bottom 0: 274.52,106.86 274.23,106.71
S$9751
  Bottom 0: 274.23,106.71 274,106.49
S$9752
  Bottom 0: 274,106.49 273.82,106.21
S$9753
  Bottom 0: 273.82,106.21 273.74,105.9
S$9754
  Bottom 0: 273.74,105.9 273.74,105.57
S$9755
  Bottom 0: 273.74,105.57 273.82,105.26
S$9756
  Bottom 0: 273.82,105.26 274,104.98
S$9757
  Bottom 0: 274,104.98 274.23,104.76
S$9758
  Bottom 0: 274.23,104.76 274.52,104.61
S$9759
  Bottom 0: 274.52,104.61 274.84,104.55
S$9760
  Bottom 0: 274.84,104.55 275.16,104.57
S$9761
  Bottom 0: 275.16,104.57 275.19,104.58
S$9762
  Bottom 0: 275.19,104.58 276.15,103.62
S$9763
  Bottom 0: 276.15,103.62 275.77,103.62
S$9764
  Bottom 0: 275.77,103.62 275.69,103.61
S$9765
  Bottom 0: 275.69,103.61 275.62,103.57
S$9766
  Bottom 0: 275.62,103.57 275.56,103.52
S$9767
  Bottom 0: 275.56,103.52 275.52,103.44
S$9768
  Bottom 0: 275.52,103.44 275.51,103.37
S$9769
  Bottom 0: 275.51,103.37 275.51,101.93
S$9770
  Bottom 0: 274.01,111.43 274.21,111.43
S$9771
  Bottom 0: 274.21,111.43 274.28,111.44
S$9772
  Bottom 0: 274.28,111.44 274.36,111.48
S$9773
  Bottom 0: 274.36,111.48 274.41,111.54
S$9774
  Bottom 0: 274.41,111.54 274.45,111.59
S$9775
  Bottom 0: 274.45,111.59 274.48,111.54
S$9776
  Bottom 0: 274.48,111.54 274.53,111.48
S$9777
  Bottom 0: 274.53,111.48 274.6,111.44
S$9778
  Bottom 0: 274.6,111.44 274.68,111.43
S$9779
  Bottom 0: 274.68,111.43 274.88,111.43
S$9780
  Bottom 0: 274.88,111.43 274.88,112.28
S$9781
  Bottom 0: 274.88,112.28 274.01,112.28
S$9782
  Bottom 0: 274.01,112.28 274.01,111.43
S$9783
  Bottom 0: 275.28,111.43 275.48,111.43
S$9784
  Bottom 0: 275.48,111.43 275.55,111.44
S$9785
  Bottom 0: 275.55,111.44 275.63,111.48
S$9786
  Bottom 0: 275.63,111.48 275.68,111.54
S$9787
  Bottom 0: 275.68,111.54 275.72,111.59
S$9788
  Bottom 0: 275.72,111.59 275.75,111.54
S$9789
  Bottom 0: 275.75,111.54 275.8,111.48
S$9790
  Bottom 0: 275.8,111.48 275.87,111.44
S$9791
  Bottom 0: 275.87,111.44 275.95,111.43
S$9792
  Bottom 0: 275.95,111.43 276.15,111.43
S$9793
  Bottom 0: 276.15,111.43 276.15,112.28
S$9794
  Bottom 0: 276.15,112.28 275.28,112.28
S$9795
  Bottom 0: 275.28,112.28 275.28,111.43
S$9796
  Bottom 0: 285.13,111.57 285.22,111.6
S$9797
  Bottom 0: 285.22,111.6 285.48,111.79
S$9798
  Bottom 0: 285.48,111.79 285.69,112.04
S$9799
  Bottom 0: 285.69,112.04 285.75,112.2
S$9800
  Bottom 0: 285.75,112.2 285.13,112.2
S$9801
  Bottom 0: 285.13,112.2 285.13,111.57
S$9802
  Bottom 0: 284.2,111.58 284.2,112.2
S$9803
  Bottom 0: 284.2,112.2 283.57,112.2
S$9804
  Bottom 0: 283.57,112.2 283.57,112.19
S$9805
  Bottom 0: 283.57,112.19 283.74,111.91
S$9806
  Bottom 0: 283.74,111.91 283.98,111.69
S$9807
  Bottom 0: 283.98,111.69 284.2,111.58
S$9808
  Bottom 0: 285.13,113.13 285.75,113.13
S$9809
  Bottom 0: 285.75,113.13 285.69,113.28
S$9810
  Bottom 0: 285.69,113.28 285.48,113.54
S$9811
  Bottom 0: 285.48,113.54 285.22,113.73
S$9812
  Bottom 0: 285.22,113.73 285.13,113.76
S$9813
  Bottom 0: 285.13,113.76 285.13,113.13
S$9814
  Bottom 0: 283.57,113.13 284.2,113.13
S$9815
  Bottom 0: 284.2,113.13 284.2,113.75
S$9816
  Bottom 0: 284.2,113.75 283.98,113.64
S$9817
  Bottom 0: 283.98,113.64 283.74,113.42
S$9818
  Bottom 0: 283.74,113.42 283.57,113.14
S$9819
  Bottom 0: 283.57,113.14 283.57,113.13
S$9820
  Bottom 0: 274.01,113.48 274.88,113.48
S$9821
  Bottom 0: 274.88,113.48 274.88,114.34
S$9822
  Bottom 0: 274.88,114.34 274.68,114.34
S$9823
  Bottom 0: 274.68,114.34 274.6,114.33
S$9824
  Bottom 0: 274.6,114.33 274.53,114.28
S$9825
  Bottom 0: 274.53,114.28 274.48,114.23
S$9826
  Bottom 0: 274.48,114.23 274.45,114.17
S$9827
  Bottom 0: 274.45,114.17 274.41,114.23
S$9828
  Bottom 0: 274.41,114.23 274.36,114.28
S$9829
  Bottom 0: 274.36,114.28 274.28,114.33
S$9830
  Bottom 0: 274.28,114.33 274.21,114.34
S$9831
  Bottom 0: 274.21,114.34 274.01,114.34
S$9832
  Bottom 0: 274.01,114.34 274.01,113.48
S$9833
  Bottom 0: 275.28,113.48 276.15,113.48
S$9834
  Bottom 0: 276.15,113.48 276.15,114.34
S$9835
  Bottom 0: 276.15,114.34 275.95,114.34
S$9836
  Bottom 0: 275.95,114.34 275.87,114.33
S$9837
  Bottom 0: 275.87,114.33 275.8,114.28
S$9838
  Bottom 0: 275.8,114.28 275.75,114.23
S$9839
  Bottom 0: 275.75,114.23 275.72,114.17
S$9840
  Bottom 0: 275.72,114.17 275.68,114.23
S$9841
  Bottom 0: 275.68,114.23 275.63,114.28
S$9842
  Bottom 0: 275.63,114.28 275.55,114.33
S$9843
  Bottom 0: 275.55,114.33 275.48,114.34
S$9844
  Bottom 0: 275.48,114.34 275.28,114.34
S$9845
